(* Logix 5000 AddOnInstructionDefinition export SetupSignVariables; software revision 17.00; part 2 of 2 *)
(* tags used below, declared in another part *)
   ENVariable3Message : BOOL;   // 0 = don't setup variable 1 = setup variable
   ENVariable4Message : BOOL;   // 0 = don't setup variable 1 = setup variable
   DN : BOOL;   // Instruction Interface Done Bit
   ER : BOOL;   // Instruction Interface Error Bit
   map_SignOutput : SINT[496];   // Ethernet/IP LEDSIGN.O Data I/O Mapping
   Packet1Sent : STRING;   // The actual packet sent to the sign (Packet1)
   Packet2Sent : STRING;   // The actual packet sent to the sign (Packet2)
   Packet3Sent : STRING;   // The actual packet sent to the sign (Packet3)
   SEQ : DINT;   // Sequence Number
   InCycle : BOOL;   // Incycle
   Error : BOOL;   // Error
   Done : BOOL;   // Done
   SignETX : STRING;   // DO NOT EDIT = ^C
   SignSOH : STRING;   // DO NOT EDIT = ^A
   SignAddress : STRING;
   SignSTX : STRING;   // DO NOT EDIT = ^B
   SignVariable4 : STRING;
   SignVariable3 : STRING;
   SignSetMemoryCommand : STRING;   // DO NOT EDIT = SM
   SignCommandCode : STRING;   // DO NOT EDIT = C
   SignSizeVariableCommand : STRING;   // DO NOT EDIT = 0010 (16 bytes of memory) enough for 16 characters
   SignFileVariableCommand : STRING;   // DO NOT EDIT = V
   TotalPacketCount : DINT[7];   // Total Character Count
   Select : DINT;   // Packet Array Select
   PacketMax : DINT;   // Max Packet Count
   Packet3Offset : DINT;
   Packet2Offset : DINT;
   Packet1Offset : DINT;
   Packet : STRING[7];   // Packet Array to send to sign
(* SetupSignVariables, continued *)

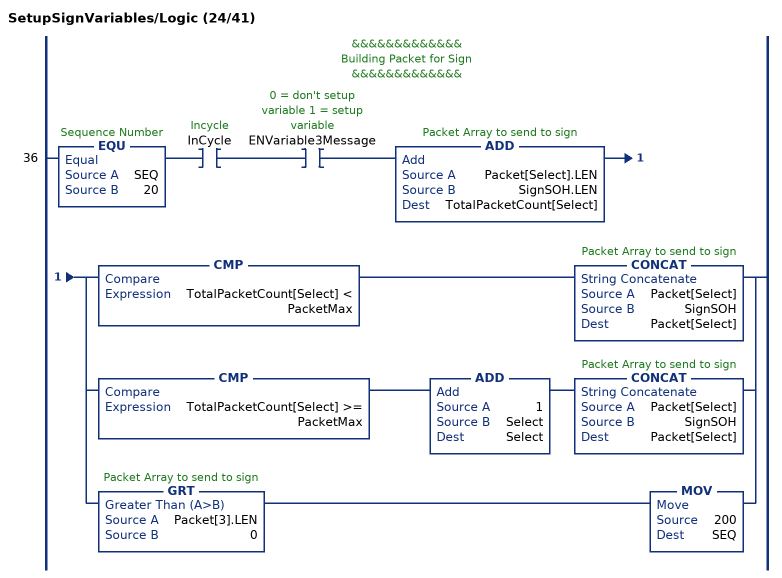
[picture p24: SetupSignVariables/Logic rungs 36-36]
   // &&&&&&&&&&&&&
   // Building Packet for Sign
   // &&&&&&&&&&&&&
   36: EQU(SEQ,20)XIC(InCycle)XIC(ENVariable3Message)ADD(Packet[Select].LEN,SignSOH.LEN,TotalPacketCount[Select])[CMP(TotalPacketCount[Select] < PacketMax) CONCAT(Packet[Select],SignSOH,Packet[Select]) ,CMP(TotalPacketCount[Select] >= PacketMax) ADD(1,Select,Select) CONCAT(Packet[Select],SignSOH,Packet[Select]) ,GRT(Packet[3].LEN,0) MOV(200,SEQ) ];
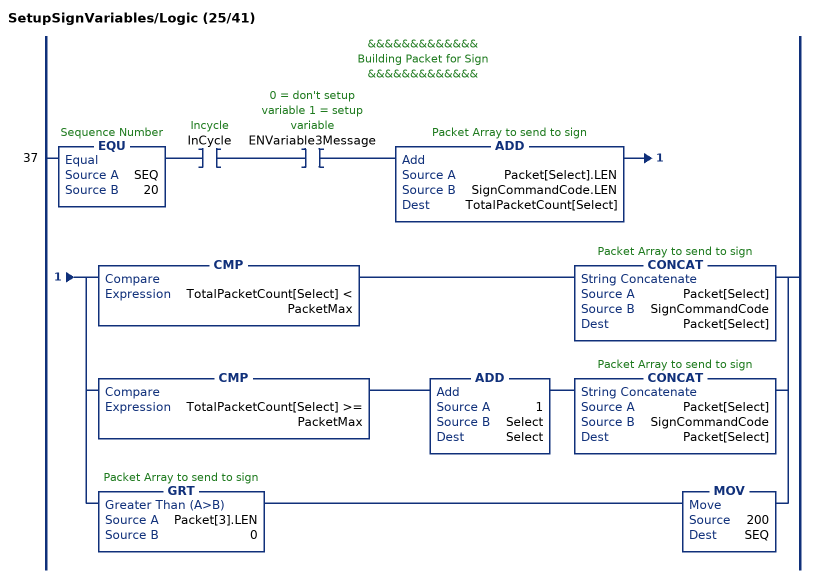
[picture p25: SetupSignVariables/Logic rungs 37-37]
   // &&&&&&&&&&&&&
   // Building Packet for Sign
   // &&&&&&&&&&&&&
   37: EQU(SEQ,20)XIC(InCycle)XIC(ENVariable3Message)ADD(Packet[Select].LEN,SignCommandCode.LEN,TotalPacketCount[Select])[CMP(TotalPacketCount[Select] < PacketMax) CONCAT(Packet[Select],SignCommandCode,Packet[Select]) ,CMP(TotalPacketCount[Select] >= PacketMax) ADD(1,Select,Select) CONCAT(Packet[Select],SignCommandCode,Packet[Select]) ,GRT(Packet[3].LEN,0) MOV(200,SEQ) ];
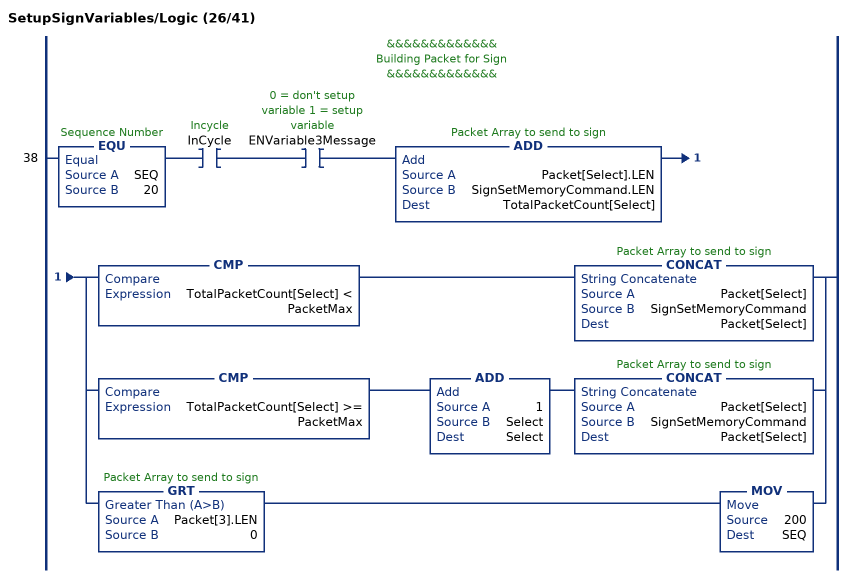
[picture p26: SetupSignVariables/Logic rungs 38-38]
   // &&&&&&&&&&&&&
   // Building Packet for Sign
   // &&&&&&&&&&&&&
   38: EQU(SEQ,20)XIC(InCycle)XIC(ENVariable3Message)ADD(Packet[Select].LEN,SignSetMemoryCommand.LEN,TotalPacketCount[Select])[CMP(TotalPacketCount[Select] < PacketMax) CONCAT(Packet[Select],SignSetMemoryCommand,Packet[Select]) ,CMP(TotalPacketCount[Select] >= PacketMax) ADD(1,Select,Select) CONCAT(Packet[Select],SignSetMemoryCommand,Packet[Select]) ,GRT(Packet[3].LEN,0) MOV(200,SEQ) ];
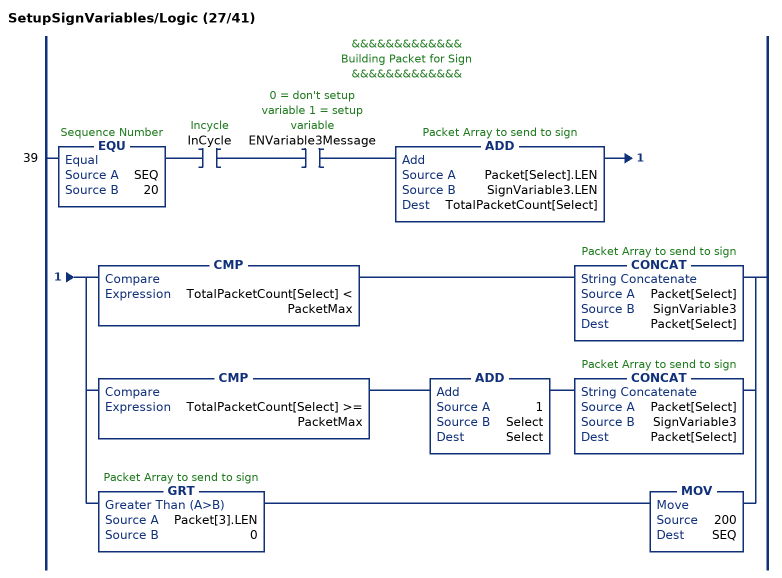
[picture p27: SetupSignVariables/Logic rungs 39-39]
   // &&&&&&&&&&&&&
   // Building Packet for Sign
   // &&&&&&&&&&&&&
   39: EQU(SEQ,20)XIC(InCycle)XIC(ENVariable3Message)ADD(Packet[Select].LEN,SignVariable3.LEN,TotalPacketCount[Select])[CMP(TotalPacketCount[Select] < PacketMax) CONCAT(Packet[Select],SignVariable3,Packet[Select]) ,CMP(TotalPacketCount[Select] >= PacketMax) ADD(1,Select,Select) CONCAT(Packet[Select],SignVariable3,Packet[Select]) ,GRT(Packet[3].LEN,0) MOV(200,SEQ) ];
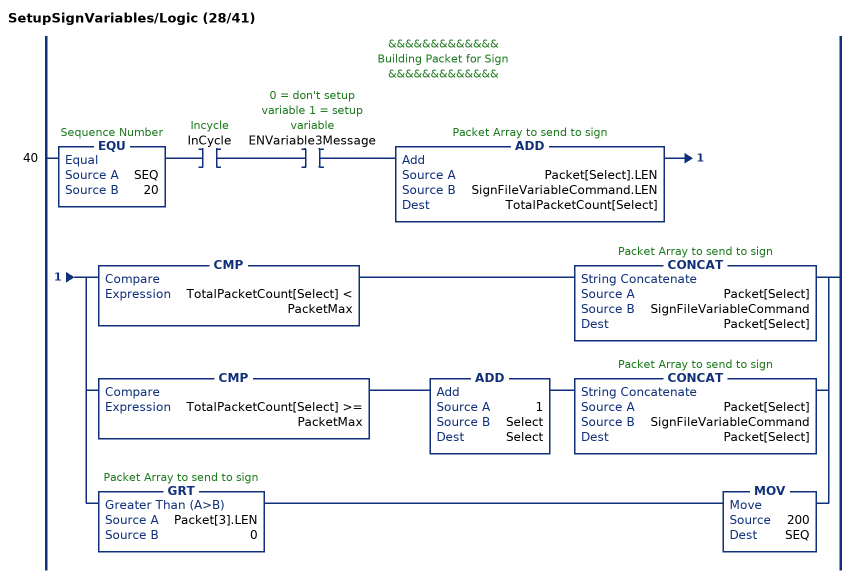
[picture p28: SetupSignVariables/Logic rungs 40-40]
   // &&&&&&&&&&&&&
   // Building Packet for Sign
   // &&&&&&&&&&&&&
   40: EQU(SEQ,20)XIC(InCycle)XIC(ENVariable3Message)ADD(Packet[Select].LEN,SignFileVariableCommand.LEN,TotalPacketCount[Select])[CMP(TotalPacketCount[Select] < PacketMax) CONCAT(Packet[Select],SignFileVariableCommand,Packet[Select]) ,CMP(TotalPacketCount[Select] >= PacketMax) ADD(1,Select,Select) CONCAT(Packet[Select],SignFileVariableCommand,Packet[Select]) ,GRT(Packet[3].LEN,0) MOV(200,SEQ) ];
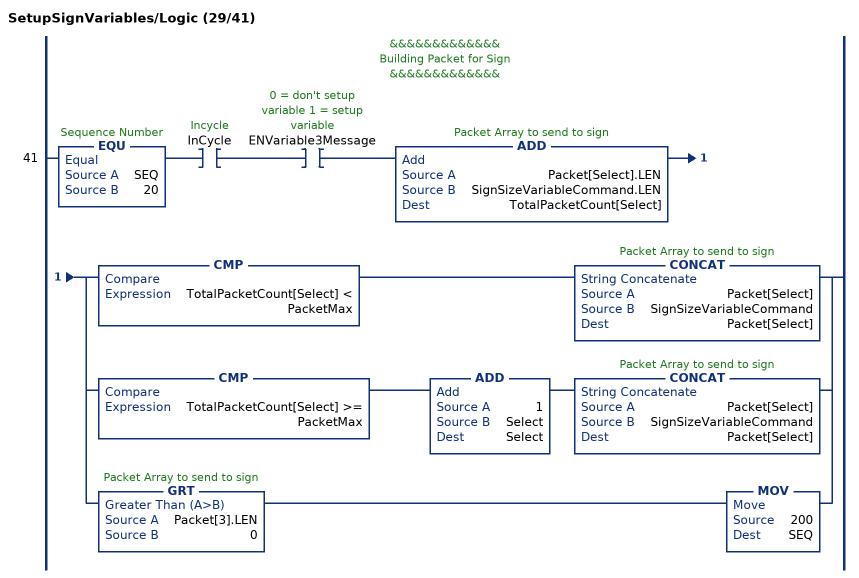
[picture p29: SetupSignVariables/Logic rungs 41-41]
   // &&&&&&&&&&&&&
   // Building Packet for Sign
   // &&&&&&&&&&&&&
   41: EQU(SEQ,20)XIC(InCycle)XIC(ENVariable3Message)ADD(Packet[Select].LEN,SignSizeVariableCommand.LEN,TotalPacketCount[Select])[CMP(TotalPacketCount[Select] < PacketMax) CONCAT(Packet[Select],SignSizeVariableCommand,Packet[Select]) ,CMP(TotalPacketCount[Select] >= PacketMax) ADD(1,Select,Select) CONCAT(Packet[Select],SignSizeVariableCommand,Packet[Select]) ,GRT(Packet[3].LEN,0) MOV(200,SEQ) ];
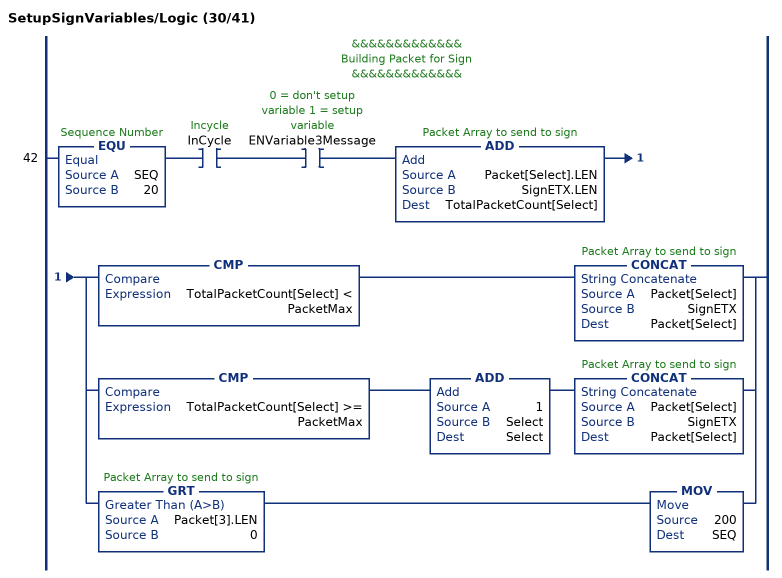
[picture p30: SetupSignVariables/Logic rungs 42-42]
   // &&&&&&&&&&&&&
   // Building Packet for Sign
   // &&&&&&&&&&&&&
   42: EQU(SEQ,20)XIC(InCycle)XIC(ENVariable3Message)ADD(Packet[Select].LEN,SignETX.LEN,TotalPacketCount[Select])[CMP(TotalPacketCount[Select] < PacketMax) CONCAT(Packet[Select],SignETX,Packet[Select]) ,CMP(TotalPacketCount[Select] >= PacketMax) ADD(1,Select,Select) CONCAT(Packet[Select],SignETX,Packet[Select]) ,GRT(Packet[3].LEN,0) MOV(200,SEQ) ];
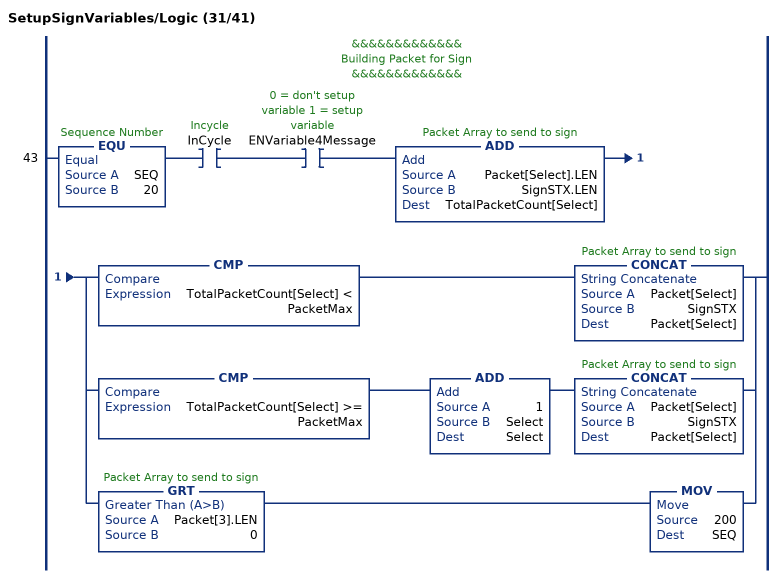
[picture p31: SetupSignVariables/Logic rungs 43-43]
   // &&&&&&&&&&&&&
   // Building Packet for Sign
   // &&&&&&&&&&&&&
   43: EQU(SEQ,20)XIC(InCycle)XIC(ENVariable4Message)ADD(Packet[Select].LEN,SignSTX.LEN,TotalPacketCount[Select])[CMP(TotalPacketCount[Select] < PacketMax) CONCAT(Packet[Select],SignSTX,Packet[Select]) ,CMP(TotalPacketCount[Select] >= PacketMax) ADD(1,Select,Select) CONCAT(Packet[Select],SignSTX,Packet[Select]) ,GRT(Packet[3].LEN,0) MOV(200,SEQ) ];
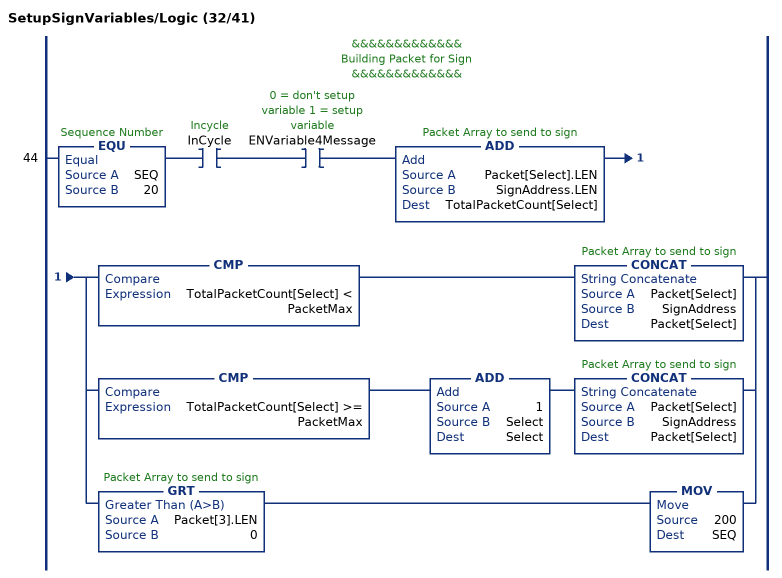
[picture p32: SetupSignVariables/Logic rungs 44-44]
   // &&&&&&&&&&&&&
   // Building Packet for Sign
   // &&&&&&&&&&&&&
   44: EQU(SEQ,20)XIC(InCycle)XIC(ENVariable4Message)ADD(Packet[Select].LEN,SignAddress.LEN,TotalPacketCount[Select])[CMP(TotalPacketCount[Select] < PacketMax) CONCAT(Packet[Select],SignAddress,Packet[Select]) ,CMP(TotalPacketCount[Select] >= PacketMax) ADD(1,Select,Select) CONCAT(Packet[Select],SignAddress,Packet[Select]) ,GRT(Packet[3].LEN,0) MOV(200,SEQ) ];
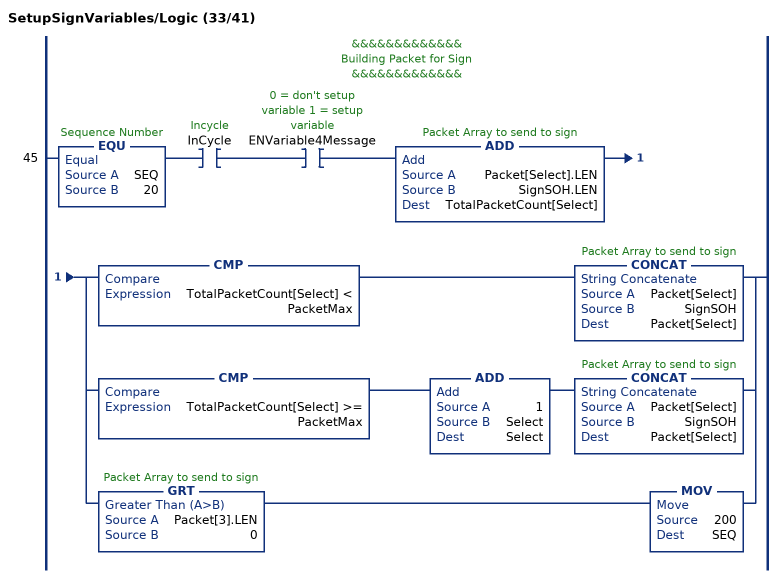
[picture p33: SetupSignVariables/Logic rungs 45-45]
   // &&&&&&&&&&&&&
   // Building Packet for Sign
   // &&&&&&&&&&&&&
   45: EQU(SEQ,20)XIC(InCycle)XIC(ENVariable4Message)ADD(Packet[Select].LEN,SignSOH.LEN,TotalPacketCount[Select])[CMP(TotalPacketCount[Select] < PacketMax) CONCAT(Packet[Select],SignSOH,Packet[Select]) ,CMP(TotalPacketCount[Select] >= PacketMax) ADD(1,Select,Select) CONCAT(Packet[Select],SignSOH,Packet[Select]) ,GRT(Packet[3].LEN,0) MOV(200,SEQ) ];
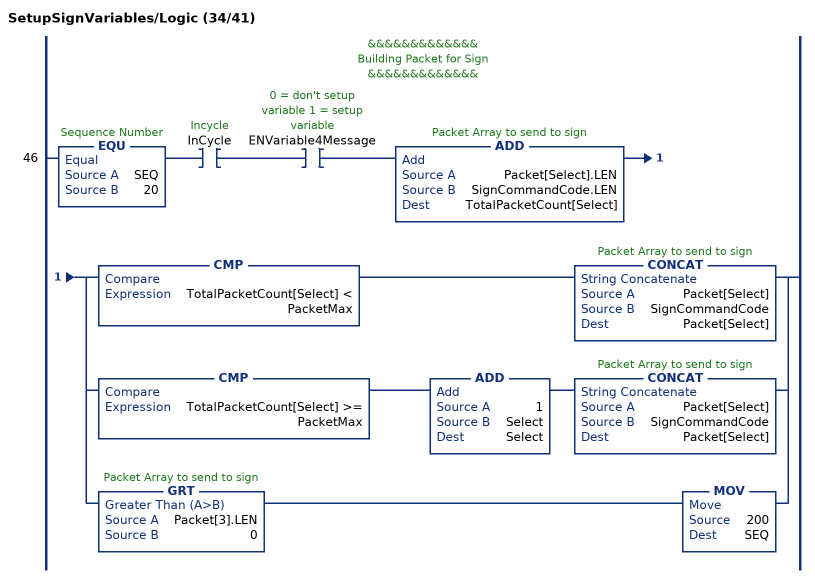
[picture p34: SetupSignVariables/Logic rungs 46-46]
   // &&&&&&&&&&&&&
   // Building Packet for Sign
   // &&&&&&&&&&&&&
   46: EQU(SEQ,20)XIC(InCycle)XIC(ENVariable4Message)ADD(Packet[Select].LEN,SignCommandCode.LEN,TotalPacketCount[Select])[CMP(TotalPacketCount[Select] < PacketMax) CONCAT(Packet[Select],SignCommandCode,Packet[Select]) ,CMP(TotalPacketCount[Select] >= PacketMax) ADD(1,Select,Select) CONCAT(Packet[Select],SignCommandCode,Packet[Select]) ,GRT(Packet[3].LEN,0) MOV(200,SEQ) ];
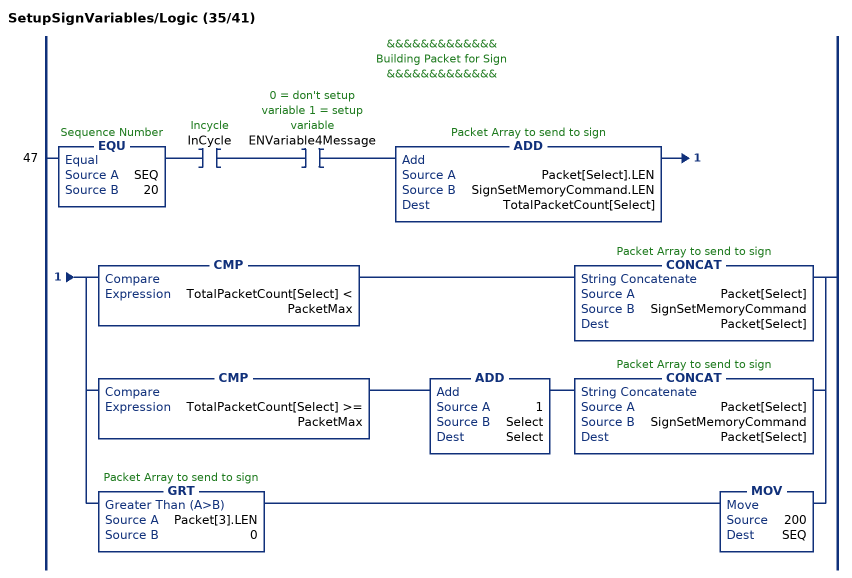
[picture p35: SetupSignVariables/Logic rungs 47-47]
   // &&&&&&&&&&&&&
   // Building Packet for Sign
   // &&&&&&&&&&&&&
   47: EQU(SEQ,20)XIC(InCycle)XIC(ENVariable4Message)ADD(Packet[Select].LEN,SignSetMemoryCommand.LEN,TotalPacketCount[Select])[CMP(TotalPacketCount[Select] < PacketMax) CONCAT(Packet[Select],SignSetMemoryCommand,Packet[Select]) ,CMP(TotalPacketCount[Select] >= PacketMax) ADD(1,Select,Select) CONCAT(Packet[Select],SignSetMemoryCommand,Packet[Select]) ,GRT(Packet[3].LEN,0) MOV(200,SEQ) ];
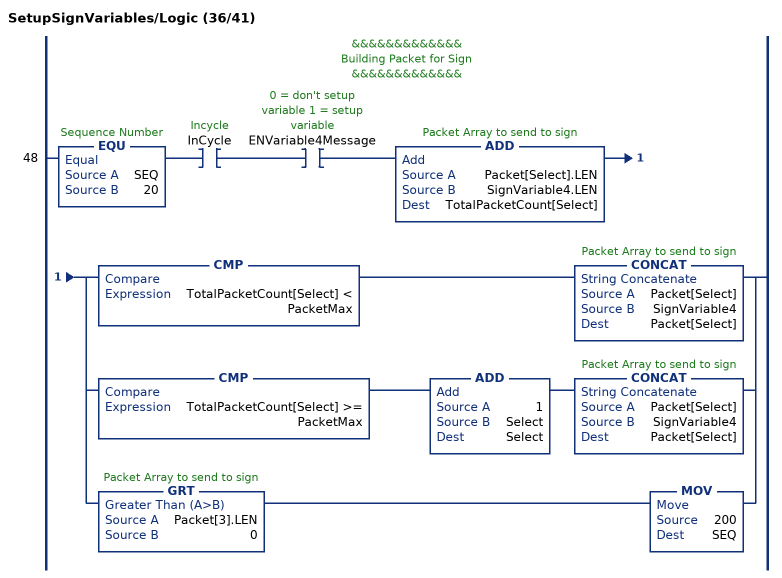
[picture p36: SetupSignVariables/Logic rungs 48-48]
   // &&&&&&&&&&&&&
   // Building Packet for Sign
   // &&&&&&&&&&&&&
   48: EQU(SEQ,20)XIC(InCycle)XIC(ENVariable4Message)ADD(Packet[Select].LEN,SignVariable4.LEN,TotalPacketCount[Select])[CMP(TotalPacketCount[Select] < PacketMax) CONCAT(Packet[Select],SignVariable4,Packet[Select]) ,CMP(TotalPacketCount[Select] >= PacketMax) ADD(1,Select,Select) CONCAT(Packet[Select],SignVariable4,Packet[Select]) ,GRT(Packet[3].LEN,0) MOV(200,SEQ) ];
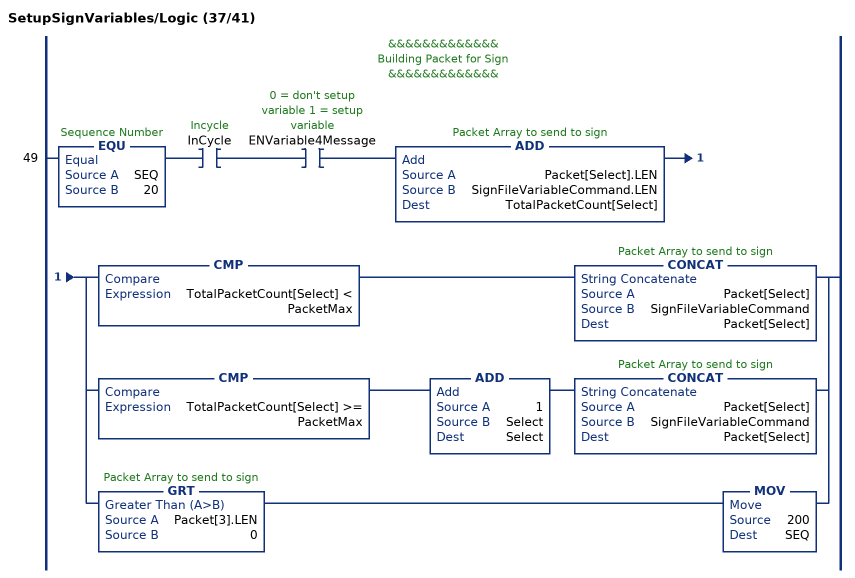
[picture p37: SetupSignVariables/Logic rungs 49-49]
   // &&&&&&&&&&&&&
   // Building Packet for Sign
   // &&&&&&&&&&&&&
   49: EQU(SEQ,20)XIC(InCycle)XIC(ENVariable4Message)ADD(Packet[Select].LEN,SignFileVariableCommand.LEN,TotalPacketCount[Select])[CMP(TotalPacketCount[Select] < PacketMax) CONCAT(Packet[Select],SignFileVariableCommand,Packet[Select]) ,CMP(TotalPacketCount[Select] >= PacketMax) ADD(1,Select,Select) CONCAT(Packet[Select],SignFileVariableCommand,Packet[Select]) ,GRT(Packet[3].LEN,0) MOV(200,SEQ) ];
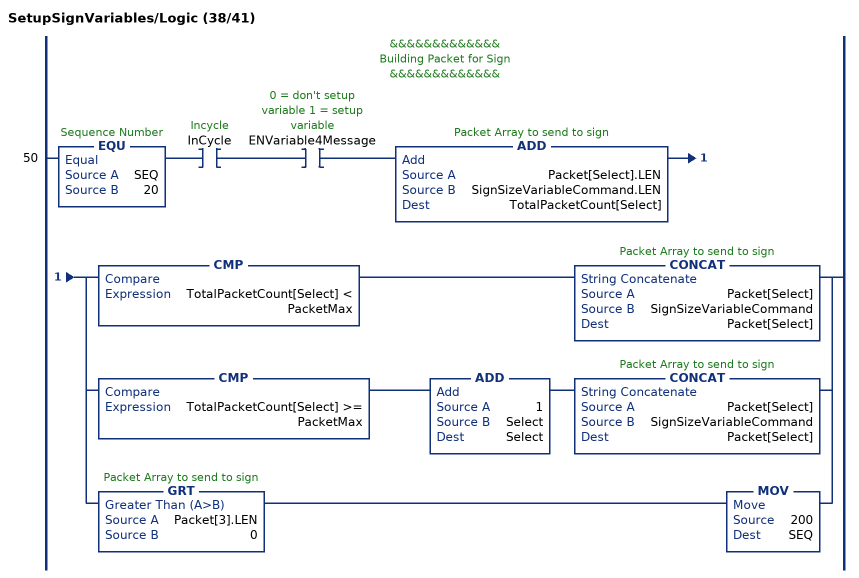
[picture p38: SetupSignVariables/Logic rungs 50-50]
   // &&&&&&&&&&&&&
   // Building Packet for Sign
   // &&&&&&&&&&&&&
   50: EQU(SEQ,20)XIC(InCycle)XIC(ENVariable4Message)ADD(Packet[Select].LEN,SignSizeVariableCommand.LEN,TotalPacketCount[Select])[CMP(TotalPacketCount[Select] < PacketMax) CONCAT(Packet[Select],SignSizeVariableCommand,Packet[Select]) ,CMP(TotalPacketCount[Select] >= PacketMax) ADD(1,Select,Select) CONCAT(Packet[Select],SignSizeVariableCommand,Packet[Select]) ,GRT(Packet[3].LEN,0) MOV(200,SEQ) ];
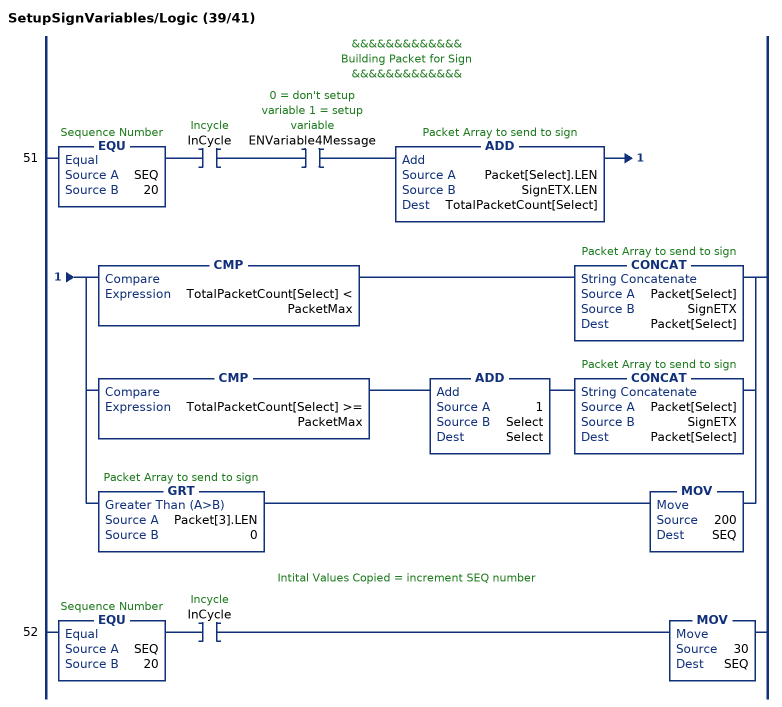
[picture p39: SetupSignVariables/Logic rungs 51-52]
   // &&&&&&&&&&&&&
   // Building Packet for Sign
   // &&&&&&&&&&&&&
   51: EQU(SEQ,20)XIC(InCycle)XIC(ENVariable4Message)ADD(Packet[Select].LEN,SignETX.LEN,TotalPacketCount[Select])[CMP(TotalPacketCount[Select] < PacketMax) CONCAT(Packet[Select],SignETX,Packet[Select]) ,CMP(TotalPacketCount[Select] >= PacketMax) ADD(1,Select,Select) CONCAT(Packet[Select],SignETX,Packet[Select]) ,GRT(Packet[3].LEN,0) MOV(200,SEQ) ];
   // Intital Values Copied = increment SEQ number
   52: EQU(SEQ,20)XIC(InCycle)MOV(30,SEQ);
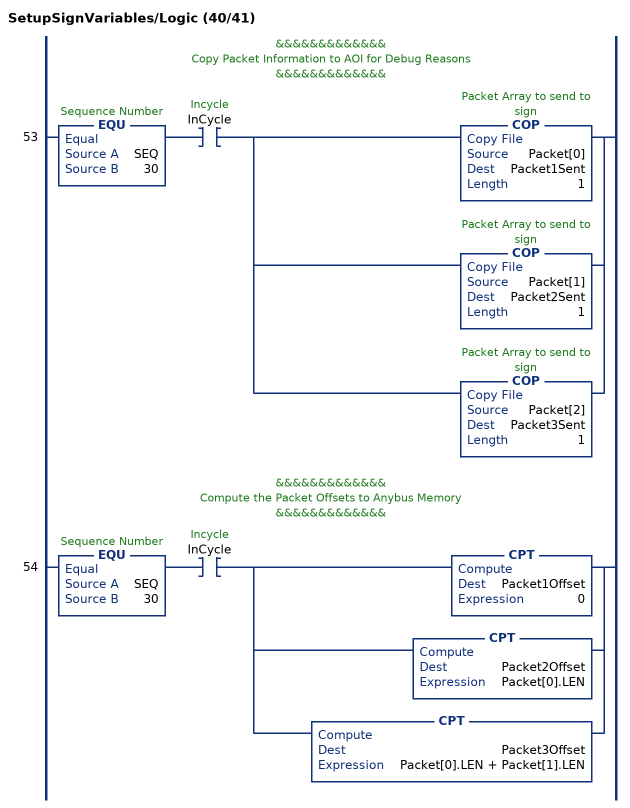
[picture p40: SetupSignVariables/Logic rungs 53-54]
   // &&&&&&&&&&&&&
   // Copy Packet Information to AOI for Debug Reasons
   // &&&&&&&&&&&&&
   53: EQU(SEQ,30)XIC(InCycle)[COP(Packet[0],Packet1Sent,1) ,COP(Packet[1],Packet2Sent,1) ,COP(Packet[2],Packet3Sent,1) ];
   // &&&&&&&&&&&&&
   // Compute the Packet Offsets to Anybus Memory
   // &&&&&&&&&&&&&
   54: EQU(SEQ,30)XIC(InCycle)[CPT(Packet1Offset,0) ,CPT(Packet2Offset,Packet[0].LEN) ,CPT(Packet3Offset,Packet[0].LEN + Packet[1].LEN) ];
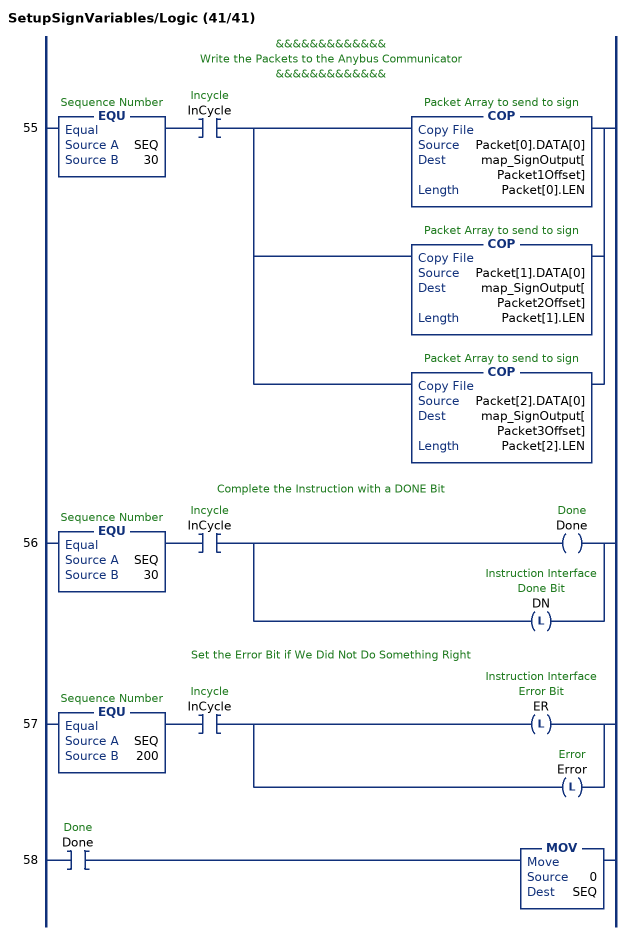
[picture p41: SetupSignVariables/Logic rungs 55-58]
   // &&&&&&&&&&&&&
   // Write the Packets to the Anybus Communicator
   // &&&&&&&&&&&&&
   55: EQU(SEQ,30)XIC(InCycle)[COP(Packet[0].DATA[0],map_SignOutput[Packet1Offset],Packet[0].LEN) ,COP(Packet[1].DATA[0],map_SignOutput[Packet2Offset],Packet[1].LEN) ,COP(Packet[2].DATA[0],map_SignOutput[Packet3Offset],Packet[2].LEN) ];
   // Complete the Instruction with a DONE Bit
   56: EQU(SEQ,30)XIC(InCycle)[OTE(Done) ,OTL(DN) ];
   // Set the Error Bit if We Did Not Do Something Right
   57: EQU(SEQ,200)XIC(InCycle)[OTL(ER) ,OTL(Error) ];
   58: XIC(Done)MOV(0,SEQ);
END_ROUTINE
END_ADD_ON_INSTRUCTION
